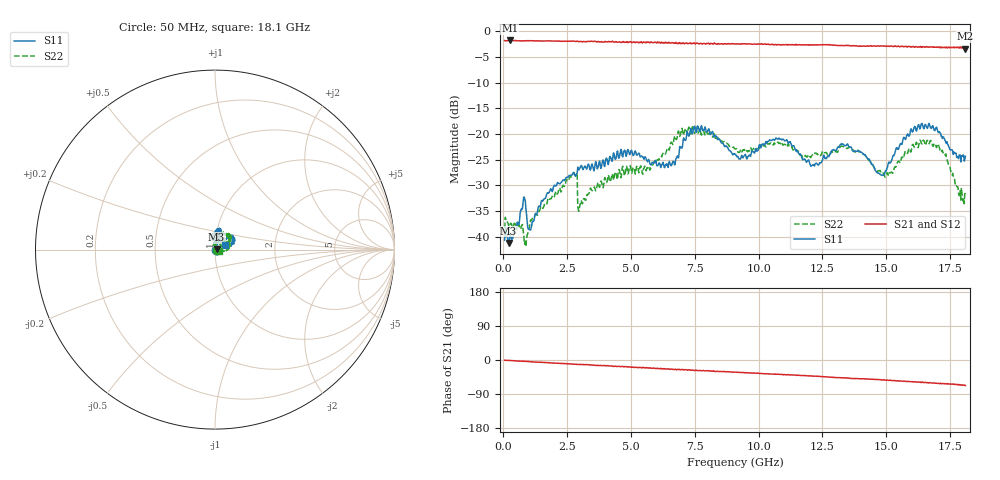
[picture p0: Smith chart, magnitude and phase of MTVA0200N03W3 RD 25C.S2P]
! Network Analyzer HP8720D.06.14 Serial No. US36140669
! 17 Jan 2005  11:51:03
! Frequency  S11  S21  S12  S22
# HZ  S  DB R 50
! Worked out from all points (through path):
!   801 points, 50 MHz to 18.1 GHz, reference 50 ohm
!   highest |S21| = -1.78 dB at 253.1 MHz (marker M1); lowest = -3.3 dB at 18.1 GHz (marker M2)
!   group delay of S21, straight-line fit = 9.76 ps
!   lowest |S11| = -41.3 dB at 207.9 MHz (marker M3), VSWR 1.02, Z = 50.9 + j0.11 ohm
!   |S11| at or under -10 dB: start of sweep to end of sweep
!   |S22| runs from -41.9 to -18.6 dB; largest |S21 - S12| = 0.026
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5e7  -40.73 -29.2  -1.80 -0.7  -1.82 -0.9  -39.96 -5.2
2.079375e8  -41.26 7.2  -1.80 -1.0  -1.81 -1.1  -37.89 -5.2
2.530625e8  -40.03 16.6  -1.78 -1.4  -1.80 -1.7  -37.75 -1.7
7.72e8  -33.34 42.3  -1.86 -3.3  -1.86 -3.6  -38.54 -31.3
9.07375e8  -35.60 6.5  -1.82 -3.9  -1.84 -4.1  -40.45 155.3
1.04275e9  -38.70 33.6  -1.81 -4.3  -1.83 -4.6  -37.55 90.6
1.787312e9  -31.45 67.7  -1.87 -7.4  -1.86 -7.5  -32.57 81.7
2.689812e9  -28.02 69.4  -1.90 -10.6  -1.91 -10.9  -28.27 86.6
3.073375e9  -26.28 69.1  -1.99 -12.1  -1.96 -12.3  -33.27 93.7
4.946062e9  -24.03 69.2  -2.07 -18.2  -2.06 -19.0  -26.37 81.4
6.074188e9  -26.07 75.5  -2.17 -23.0  -2.18 -23.0  -25.13 78.2
6.660812e9  -25.34 68.1  -2.30 -24.6  -2.27 -24.4  -21.77 76.4
7.54075e9  -19.58 73.7  -2.35 -26.4  -2.19 -28.0  -18.65 47.3
9.075e9  -23.95 92.3  -2.45 -32.0  -2.43 -32.3  -22.92 25.8
1.076719e10  -21.00 93.2  -2.58 -37.8  -2.63 -38.2  -21.60 23.1
1.209838e10  -26.13 81.3  -2.62 -42.3  -2.63 -42.6  -24.16 38.3
1.327162e10  -21.97 52.4  -2.75 -46.9  -2.77 -47.4  -22.40 43.3
1.476075e10  -27.92 45.3  -2.86 -51.8  -2.86 -52.4  -27.13 28.7
1.509919e10  -25.47 20.3  -2.91 -53.9  -2.84 -54.0  -28.14 40.1
1.604681e10  -19.52 23.5  -2.95 -57.5  -3.07 -57.7  -22.04 29.5
1.667856e10  -17.95 36.2  -3.11 -60.2  -3.00 -60.4  -21.91 14.3
1.81e10  -24.35 27.2  -3.35 -67.2  -3.26 -68.2  -31.73 -15.5
